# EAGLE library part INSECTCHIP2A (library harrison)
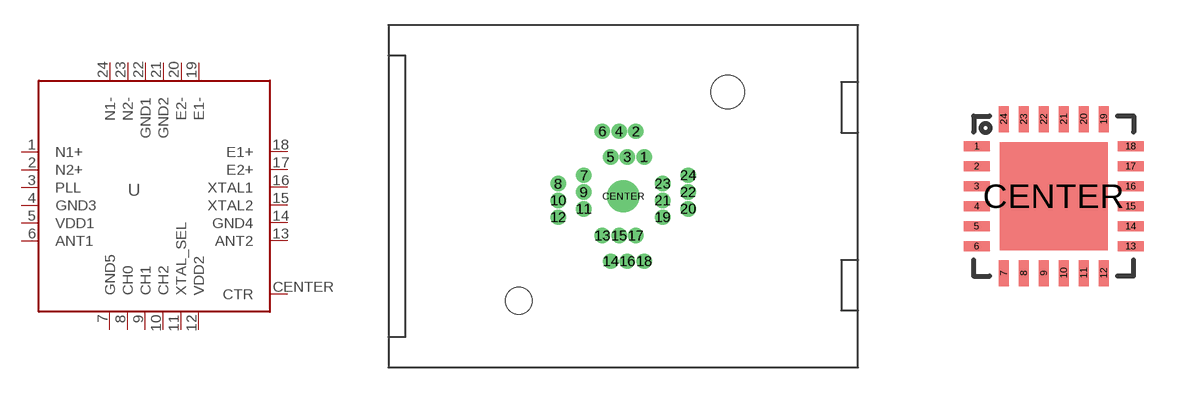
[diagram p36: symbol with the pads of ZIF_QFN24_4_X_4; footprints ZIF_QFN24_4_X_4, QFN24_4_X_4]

Designator prefix U

## INSECTCHIP2AZIF  [ZIF_QFN24_4_X_4]
1  N1+  in
2  N2+  in
3  PLL  pas
4  GND3  pwr
5  VDD1  pwr
6  ANT1  pas
7  GND5  pwr
8  CH0  in
9  CH1  in
10  CH2  in
11  XTAL_SEL  in
12  VDD2  pwr
13  ANT2  pas
14  GND4  pwr
15  XTAL2  pas
16  XTAL1  pas
17  E2+  in
18  E1+  in
19  E1-  in
20  E2-  in
21  GND2  pwr
22  GND1  pwr
23  N2-  in
24  N1-  in
CENTER  CTR  pwr

## INSECTCHIP2AQFN  [QFN24_4_X_4]
Pads as for ZIF_QFN24_4_X_4

## Footprint ZIF_QFN24_4_X_4 (pad centres in mm)
drill 0.41 pad 0.813: 1 1.25,2.35; 2 0.75,3.875; 3 0.25,2.35; 4 -0.25,3.875; 5 -0.75,2.35; 6 -1.25,3.875; 7 -2.35,1.25; 8 -3.875,0.75; 9 -2.35,0.25; 10 -3.875,-0.25; 11 -2.35,-0.75; 12 -3.875,-1.25; 13 -1.25,-2.35; 14 -0.75,-3.875; 15 -0.25,-2.35; 16 0.25,-3.875; 17 0.75,-2.35; 18 1.25,-3.875; 19 2.35,-1.25; 20 3.875,-0.75; 21 2.35,-0.25; 22 3.875,0.25; 23 2.35,0.75; 24 3.875,1.25
drill 1.02 pad 1.93: CENTER 0,0
hole 1.6 at -6.23,-6.23
hole 2 at 6.22,6.22

## Footprint QFN24_4_X_4 (pad centres in mm)
smd 0.65 x 0.25: 1 -1.925,1.25; 2 -1.925,0.75; 3 -1.925,0.25; 4 -1.925,-0.25; 5 -1.925,-0.75; 6 -1.925,-1.25; 13 1.925,-1.25; 14 1.925,-0.75; 15 1.925,-0.25; 16 1.925,0.25; 17 1.925,0.75; 18 1.925,1.25
smd 0.25 x 0.65: 7 -1.25,-1.925; 8 -0.75,-1.925; 9 -0.25,-1.925; 10 0.25,-1.925; 11 0.75,-1.925; 12 1.25,-1.925; 19 1.25,1.925; 20 0.75,1.925; 21 0.25,1.925; 22 -0.25,1.925; 23 -0.75,1.925; 24 -1.25,1.925
smd 2.7 x 2.7: CENTER 0,0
